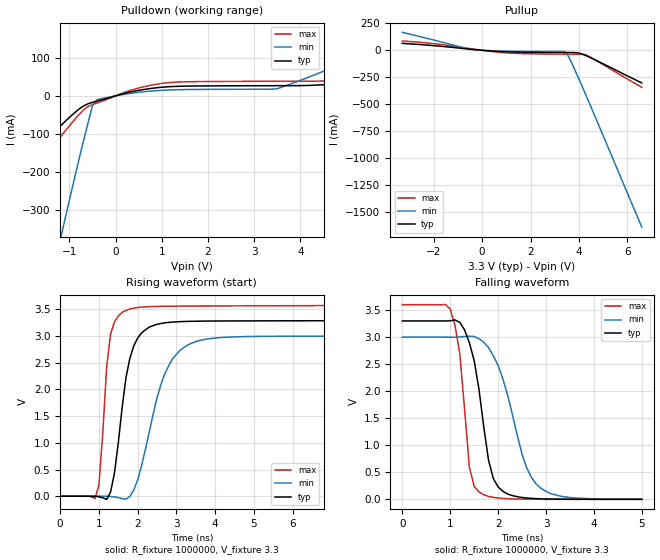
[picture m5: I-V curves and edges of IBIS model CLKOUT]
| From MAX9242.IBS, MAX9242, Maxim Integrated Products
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|   Model CLKOUT
[Model]   CLKOUT
Model_type   Output
|Signal   RxCLKOUT
|   typ   min   max
C_comp   3.1pF   2.8pF   3.3pF
[Temperature Range]   25.00   85.00   -40
[Voltage Range]   3.30V   3.00V   3.60V
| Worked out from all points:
|   slope of the pulldown table from 0 to 0.495 V, typ, clamps not added: 34.5 ohm
|   slope of the pullup table from 0 to 0.495 V, typ, clamps not added: 59.6 ohm
|   falling waveform, R_fixture 1000000, V_fixture 3.3: 20-80 % time 341ps typ, 560ps min, 223ps max; typ from 3.3 V to 0 V
|   rising waveform, R_fixture 1000000, V_fixture 3.3: 20-80 % time 382ps typ, 662ps min, 221ps max; typ from 0 V to 3.29 V
[Pulldown]
|Volts   I(typ)   I(min)   I(max)
-3.3V     -318.4mA   -1.5A      -391.2mA
-3V       -285.9mA   -1.341A    -353.2mA
-1.2V     -79.68mA   -379.3mA   -108.2mA
-1.1V     -67.98mA   -326.4mA   -93.39mA
-700mV    -26.87mA   -120.7mA   -37.61mA
-500mV    -17.02mA   -25.34mA   -22.92mA
-400mV    -13.74mA   -9.961mA   -18.69mA
200mV     6.7mA      4.386mA    9.474mA
1.2V      24.36mA    15.67mA    35.29mA
3.5V      26.74mA    18.85mA    38.31mA
4.9V      33.47mA    84.9mA     43.08mA
6.6V      63.01mA    178.2mA    82.36mA
[Pullup]
|Volts   I(typ)   I(min)   I(max)
-3.3V     64.23mA    167.1mA    86.59mA
-1.9V     41.34mA    89.58mA    59.51mA
-500mV    10.34mA    8.176mA    16.33mA
1.2V      -15.58mA   -9.34mA    -26.82mA
3.4V      -20.81mA   -12.5mA    -36.09mA
3.5V      -20.91mA   -25.88mA   -36.23mA
4V        -25.8mA    -266.4mA   -36.89mA
4.3V      -50.19mA   -421.9mA   -45.18mA
6.6V      -303.6mA   -1.645A    -344.8mA
[Ramp]
|Variable   typ   min   max
dV/dt_r  1.91/0.36n  1.80/0.66n  2.03/0.20n
dV/dt_f  1.96/0.32n  1.79/0.54n  2.25/0.22n
R_load=1000000
[Falling Waveform]
R_fixture = 1000000
C_fixture = 0.0
V_fixture = 3.3
V_fixture_min = 3.0
V_fixture_max = 3.6
|Time   V(typ)   V(min)   V(max)
0s        3.3V       3V         3.6V
1ns       3.302V     2.999V     3.521V
1.2ns     3.273V     3.004V     2.697V
1.4ns     2.898V     3.018V     591.7mV
1.6ns     2.04V      2.972V     137.4mV
1.8ns     724.4mV    2.807V     53.33mV
1.9ns     386.2mV    2.658V     36.56mV
2.5ns     33.83mV    832.8mV    3.974mV
2.8ns     12.86mV    279.2mV    1.538mV
5ns       53.98uV    1.168mV    9.818uV
[Rising Waveform]
R_fixture = 1000000
C_fixture = 0.0
V_fixture = 3.3
V_fixture_min = 3.0
V_fixture_max = 3.6
|Time   V(typ)   V(min)   V(max)
0s        0V         0V         0V
900ps     -39.17uV   -101.6uV   -41.36mV
1ns       -9.565mV   368.5uV    206.6mV
1.2ns     -58.01mV   -78.28uV   2.413V
1.3ns     73.47mV    -4.509mV   3.032V
1.8ns     2.582V     -2.877mV   3.504V
2.1ns     3.054V     567.6mV    3.539V
2.7ns     3.245V     2.288V     3.555V
3.7ns     3.277V     2.931V     3.56V
20ns      3.294V     2.997V     3.588V
